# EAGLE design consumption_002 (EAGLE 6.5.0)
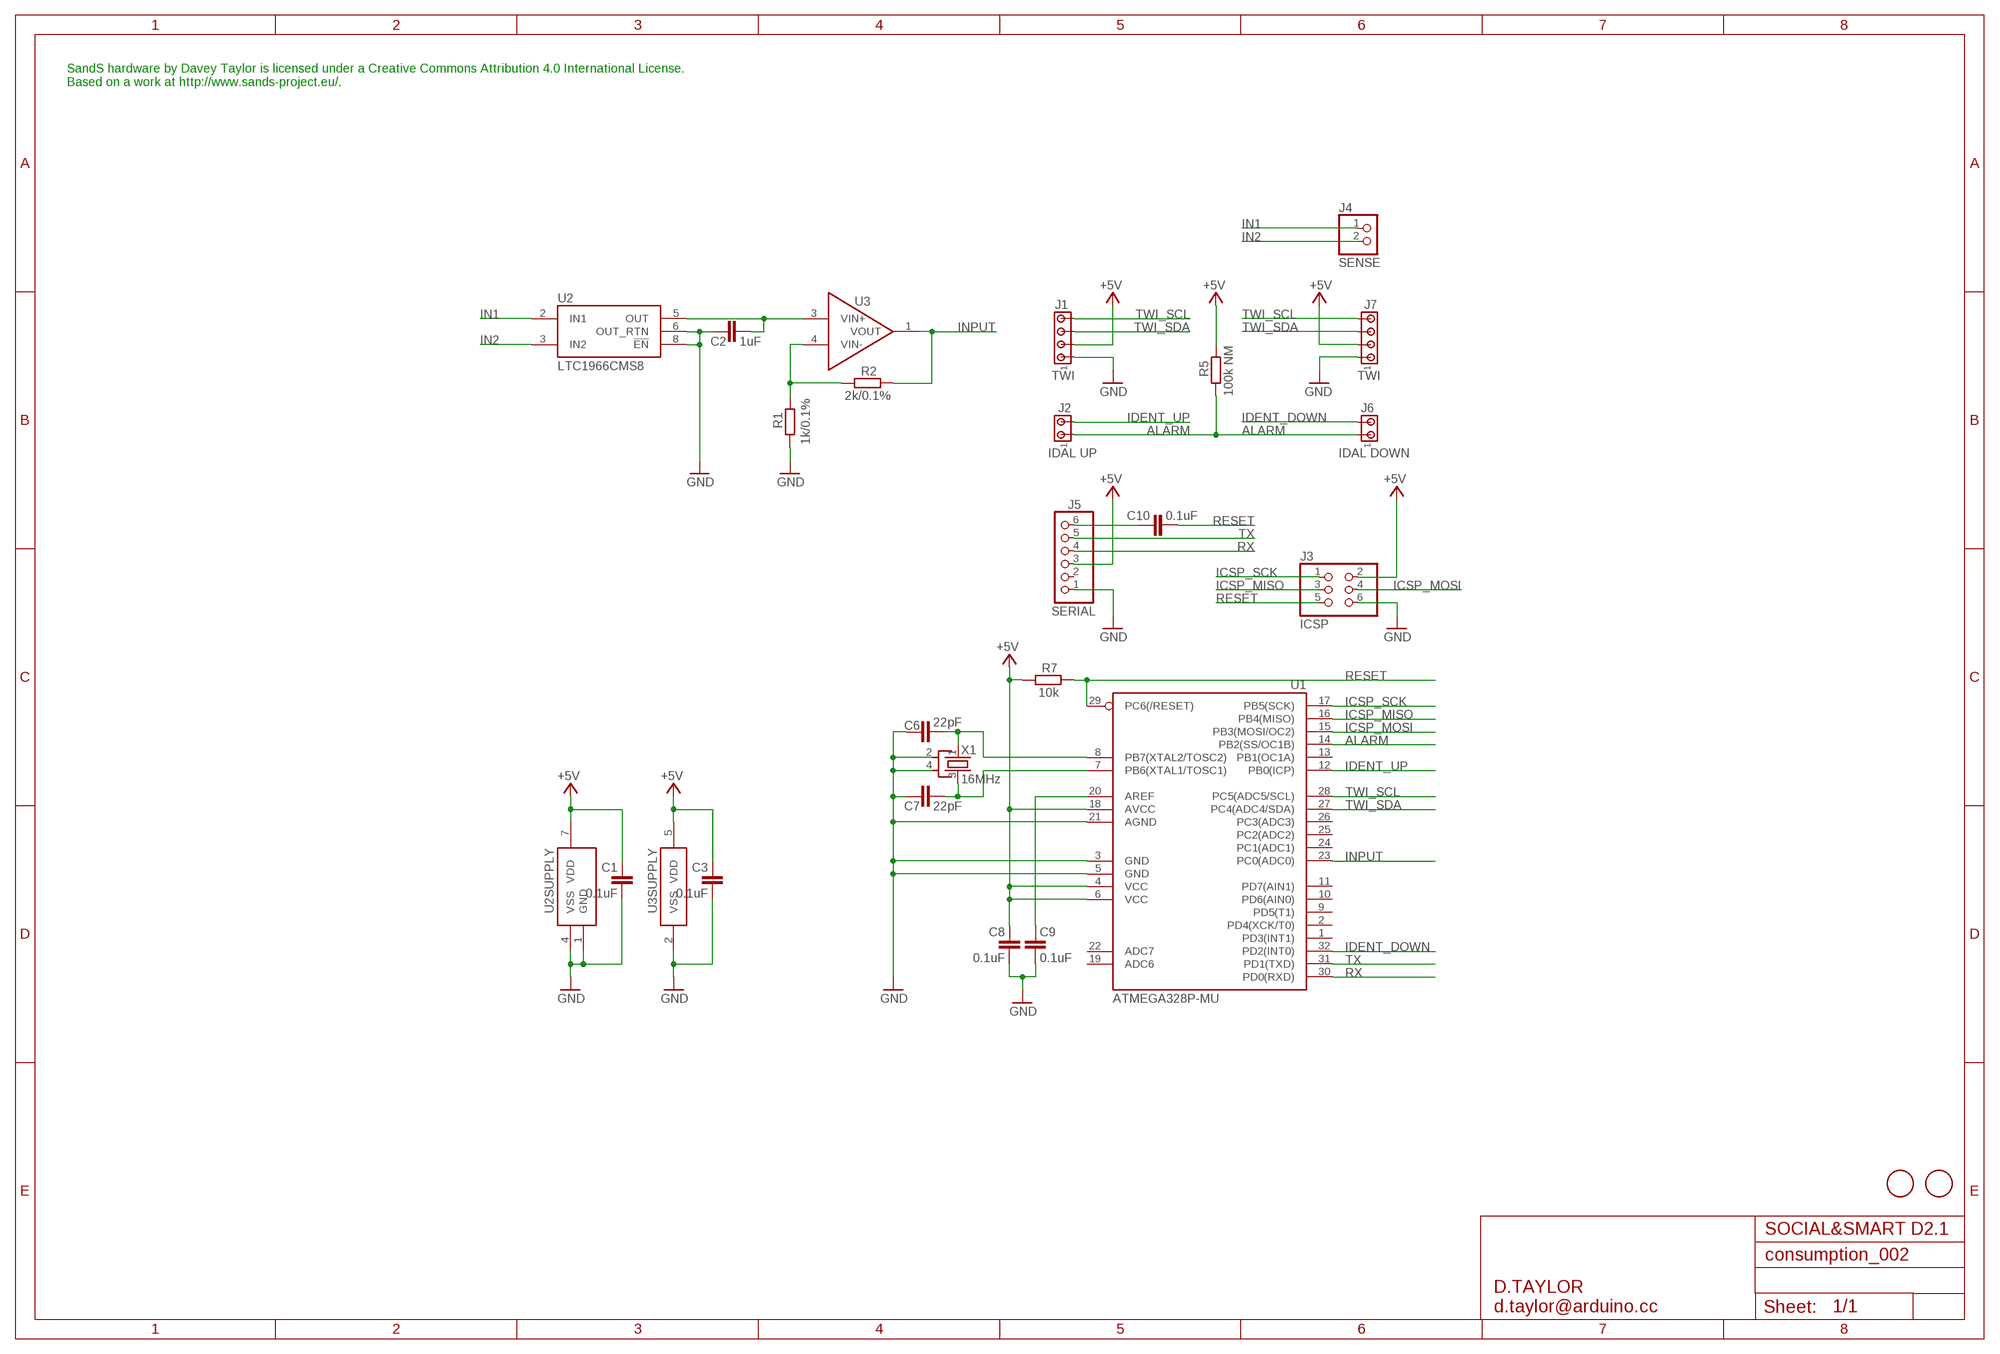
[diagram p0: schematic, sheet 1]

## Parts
C1  0.1uF  C-EUC0603  [C0603]
C2  1uF  C-EUC0603  [C0603]
C3  0.1uF  C-EUC0603  [C0603]
C6  22pF  C-EUC0603  [C0603]
C7  22pF  C-EUC0603  [C0603]
C8  0.1uF  C-EUC0603  [C0603]
C9  0.1uF  C-EUC0603  [C0603]
C10  0.1uF  C-EUC0603  [C0603]
J1  TWI  MTA04-100  [10X04MTA]
J2  IDAL UP  MTA02-100  [10X02MTA]
J3  ICSP  PINHD-2X3  [2X03]
J4  SENSE  MKDS_1,5/2-5,08  [MKDS1,5/2-5,08]
J5  SERIAL  PINHD-1X6  [1X06]
J6  IDAL DOWN  MTA02-100  [10X02MTA]
J7  TWI  MTA04-100  [10X04MTA]
R1  1k/0.1%  R-EU_R0603  [R0603]
R2  2k/0.1%  R-EU_R0603  [R0603]
R5  100k NM  R-EU_R0603  [R0603]
R7  10k  R-EU_R0603  [R0603]
U1  ATMEGA328P-MU  [MLF32-M1-A]
U2  LTC1966CMS8  [MSOP08]
U3  MCP6401T-E/OT  MCP6401-E/OT  [SOT-23-5]
U$5  FIDUCIALMOUNT  [FIDUCIA-MOUNT]
U$6  FIDUCIALMOUNT  [FIDUCIA-MOUNT]
X1  16MHz  CRYSTAL-KX7  [XTAL-3.2-2.5]

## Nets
+5V: C1.1 C3.1 C8.1 J1.2 J3.2 J5.3 J7.2 R5.2 R7.1 U1.4(VCC) U1.6(VCC) U1.18(AVCC) U2.7(VDD) U3.5(VDD)
ALARM: J2.1 J6.1 R5.1 U1.14(PB2(SS/OC1B))
GND: C1.2 C2.1 C3.2 C6.1 C7.1 C8.2 C9.2 J1.1 J3.6 J5.1 J7.1 R1.1 U1.3(GND) U1.5(GND) U1.21(AGND) U2.1(GND) U2.4(VSS) U2.6(OUT_RTN) U2.8(!EN!) U3.2(VSS) X1.2(SH1) X1.4(SH2)
ICSP_MISO: J3.3 U1.16(PB4(MISO))
ICSP_MOSI: J3.4 U1.15(PB3(MOSI/OC2))
ICSP_SCK: J3.1 U1.17(PB5(SCK))
IDENT_DOWN: J6.2 U1.32(PD2(INT0))
IDENT_UP: J2.2 U1.12(PB0(ICP))
IN1: J4.1 U2.2(IN1)
IN2: J4.2 U2.3(IN2)
INPUT: R2.1 U1.23(PC0(ADC0)) U3.1(VOUT)
N$1: C2.2 U2.5(OUT) U3.3(VIN+)
N$2: R1.2 R2.2 U3.4(VIN-)
N$3: C9.1 U1.20(AREF)
N$6: C6.2 U1.8(PB7(XTAL2/TOSC2)) X1.1(X1)
N$7: C7.2 U1.7(PB6(XTAL1/TOSC1)) X1.3(X2)
N$9: C10.1 J5.6
RESET: C10.2 J3.5 R7.2 U1.29(PC6(/RESET))
RX: J5.4 U1.30(PD0(RXD))
TWI_SCL: J1.4 J7.4 U1.28(PC5(ADC5/SCL))
TWI_SDA: J1.3 J7.3 U1.27(PC4(ADC4/SDA))
TX: J5.5 U1.31(PD1(TXD))
Unconnected: J5.2 U1.1(PD3(INT1)) U1.2(PD4(XCK/T0)) U1.9(PD5(T1)) U1.10(PD6(AIN0)) U1.11(PD7(AIN1)) U1.13(PB1(OC1A)) U1.19(ADC6) U1.22(ADC7) U1.24(PC1(ADC1)) U1.25(PC2(ADC2)) U1.26(PC3(ADC3))

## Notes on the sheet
- SandS hardware by Davey Taylor is licensed under a Creative Commons Attribution 4.0 International License.
  Based on a work at http://www.sands-project.eu/.
- SOCIAL&SMART D2.1
- D.TAYLOR
  d.taylor@arduino.cc

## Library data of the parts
C1-C3 C6-C10 = rcl:C-EU: CAPACITOR, European symbol
J1 J7 = con-amp:MTA04-100: AMP connector
J2 J6 = con-amp:MTA02-100: AMP connector
J3 = pinhead:PINHD-2X3: PIN HEADER
J4 = d_taylor:MKDS_1,5/2-5,08: Screw terminal header
J5 = pinhead:PINHD-1X6: PIN HEADER
R1 R2 R5 R7 = rcl:R-EU_: RESISTOR, European symbol
U1 = d_taylor:ATMEGA*: MICROCONTROLLER 8 Kbytes FLASH 1 kbytes SRAM 512 bytes EEPROM USART 6-channel 10 bit ADC 2-channel 8 bit ADC Source: avr.lbr
U2 = d_taylor:LTC1966*MS8: Precision Micropower Delta-Sigma RMS-to-DC Converter
U3 = d_taylor:MCP6401*
U$5 U$6 = SmartPrj:FIDUCIALMOUNT
X1 = d_taylor:CRYSTAL-KX7

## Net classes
1 PWR: width 0.406 mm, clearance 0.254 mm

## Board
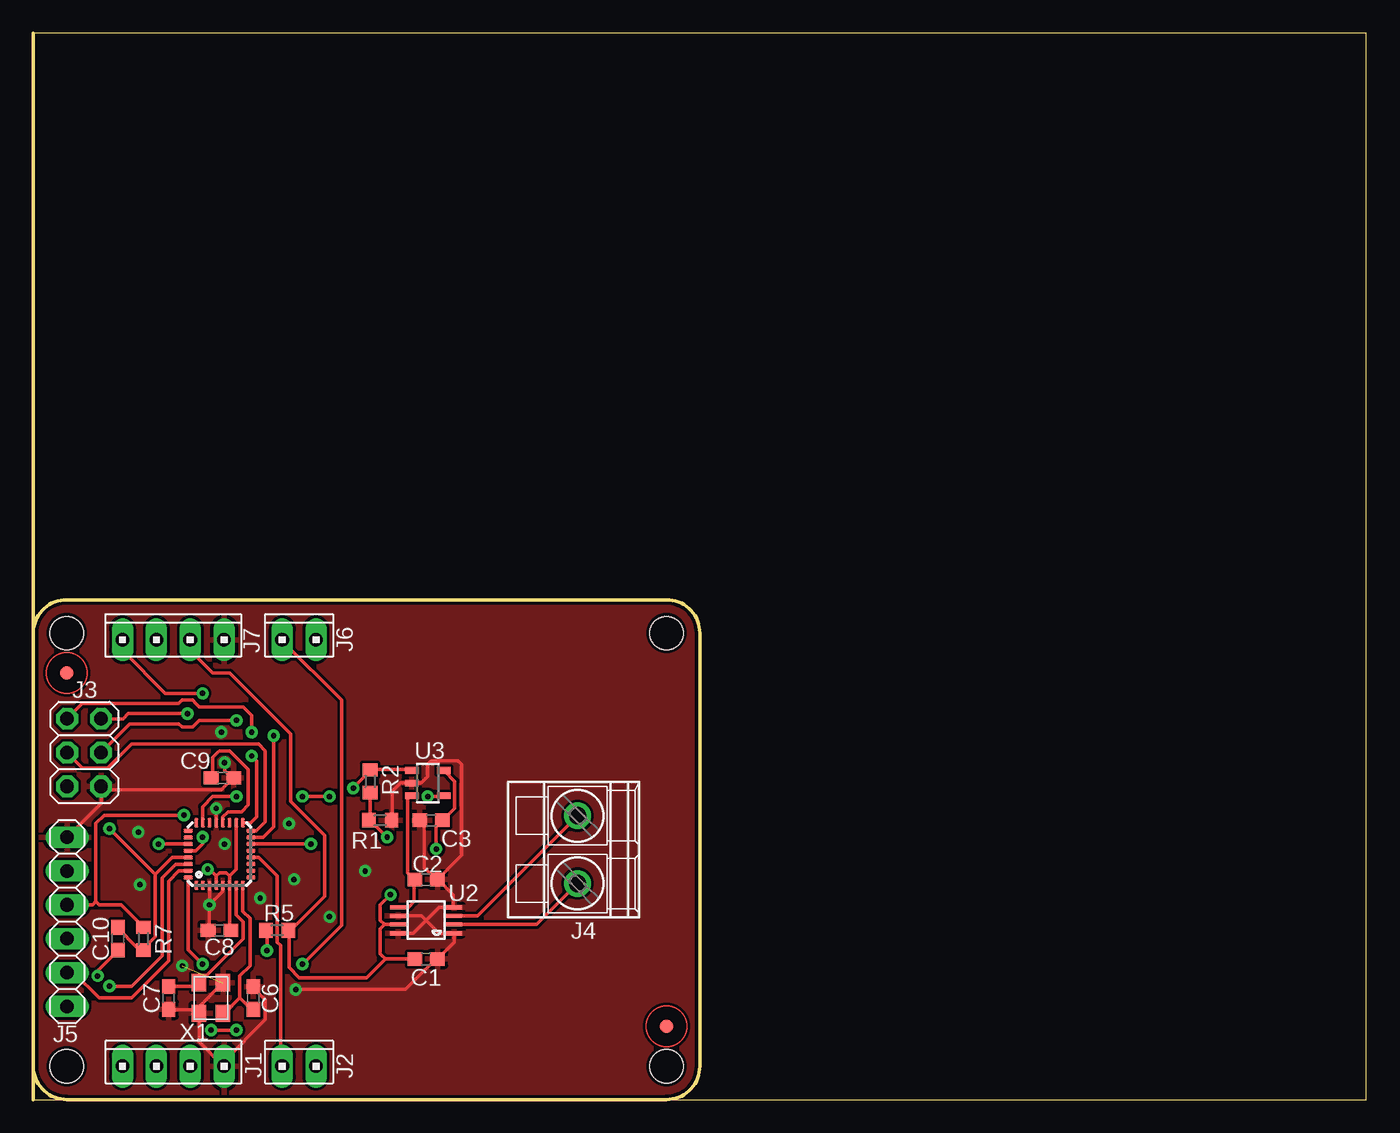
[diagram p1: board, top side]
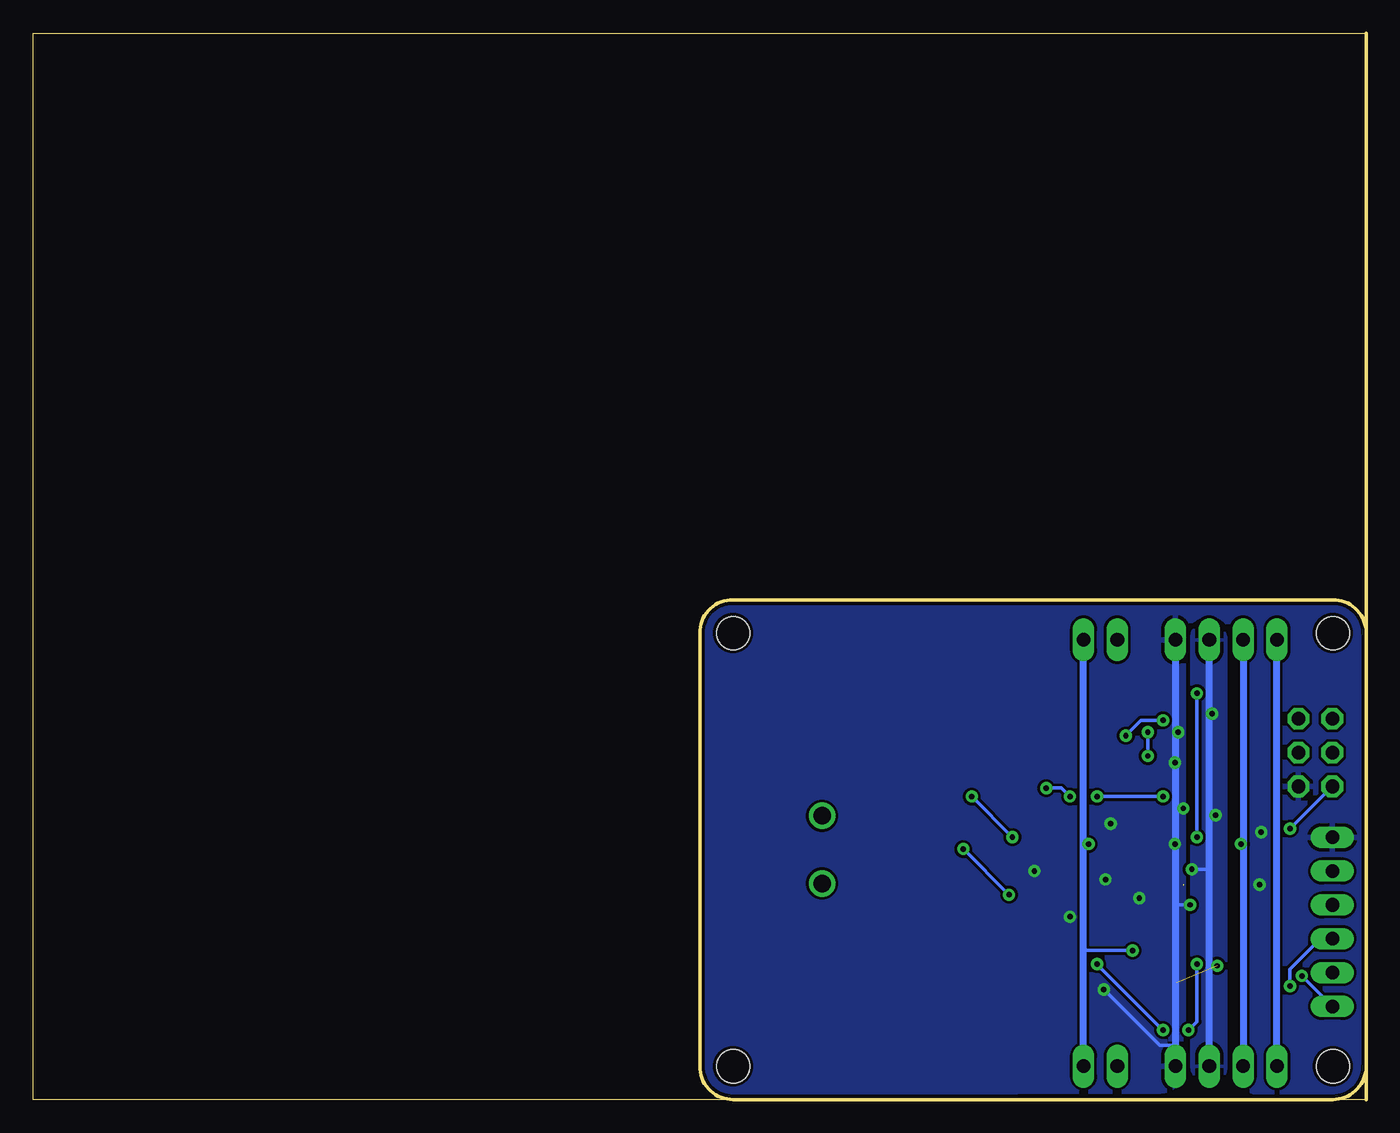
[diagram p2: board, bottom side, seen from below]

Size 100 x 80 mm. Coordinates in mm from the lower left corner, seen from the top.
Outline: 0,35 0,80 100,80 100,0 0,0 0,35
Outline: 0,35 arc-90 2.5,37.5 47.5,37.5 arc-90 50,35 50,2.5 arc-90 47.5,0 2.5,0 arc-90 0,2.5 0,35
Copper layers (1*16): Top 0.035mm / dielectric 1.5mm / Bottom 0.035mm
Design rules "smartprj-mini *": minimum track width 8mil, minimum drill 16mil, track to track 8mil, track to pad 8mil, pad to pad 0.200659375mm, via to via 8mil, smd to smd 4mil, copper to edge 10mil, drill to drill 8mil, minimum pad ring 12mil, minimum via ring 10mil, stop-mask expansion 2mil, vias tented up to drill 20mil, thermal gap 10mil
Holes 2.5 mm at 2.5,35 2.5,2.5 47.5,2.5 47.5,35

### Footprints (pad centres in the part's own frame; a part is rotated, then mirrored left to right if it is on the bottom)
C0603 = smd 1.1 x 1: 1 -0.85,0; 2 0.85,0
10X04MTA = drill 1.016 long: 1 3.81,0; 2 1.27,0; 3 -1.27,0; 4 -3.81,0
10X02MTA = drill 1.016 long: 1 1.27,0; 2 -1.27,0
2X03 = drill 1.016 octagon: 1 -2.54,-1.27; 2 -2.54,1.27; 3 0,-1.27; 4 0,1.27; 5 2.54,-1.27; 6 2.54,1.27
MKDS1,5/2-5,08 = drill 1.3 pad 2: 1 -2.54,0; 2 2.54,0
1X06 = drill 1.016 long: 1 -6.35,0; 2 -3.81,0; 3 -1.27,0; 4 1.27,0; 5 3.81,0; 6 6.35,0
R0603 = smd 1 x 1.1: 1 -0.85,0; 2 0.85,0
MLF32-M1-A = smd 0.7 x 0.3: 1 -2.35,1.75; 2 -2.35,1.25; 3 -2.35,0.75; 4 -2.35,0.25; 5 -2.35,-0.25; 6 -2.35,-0.75; 7 -2.35,-1.25; 8 -2.35,-1.75; 17 2.35,-1.75; 18 2.35,-1.25; 19 2.35,-0.75; 20 2.35,-0.25; 21 2.35,0.25; 22 2.35,0.75; 23 2.35,1.25; 24 2.35,1.75 | smd 0.3 x 0.7: 9 -1.75,-2.35; 10 -1.25,-2.35; 11 -0.75,-2.35; 12 -0.25,-2.35; 13 0.25,-2.35; 14 0.75,-2.35; 15 1.25,-2.35; 16 1.75,-2.35; 25 1.75,2.35; 26 1.25,2.35; 27 0.75,2.35; 28 0.25,2.35; 29 -0.25,2.35; 30 -0.75,2.35; 31 -1.25,2.35; 32 -1.75,2.35
MSOP08 = smd 0.3 x 1.2: 1 -0.976,-2.113; 2 -0.326,-2.113; 3 0.324,-2.113; 4 0.974,-2.113; 5 0.974,2.112; 6 0.324,2.112; 7 -0.326,2.112; 8 -0.976,2.112
SOT-23-5 = smd 0.5 x 1: 1 -0.95,-1.2; 2 0,-1.2; 3 0.95,-1.2; 4 0.95,1.2; 5 -0.95,1.2
FIDUCIA-MOUNT = smd 1.016 x 1.016: P$1 0,0
XTAL-3.2-2.5 = smd 1.3 x 1.1: 1 -1.15,-0.9; 2 1.15,-0.9; 3 1.15,0.9; 4 -1.15,0.9

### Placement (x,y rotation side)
C1  29.46,10.54 0 top
C2  29.46,16.51 180 top
C3  29.84,20.95 180 top
C6  16.51,7.62 270 top
C7  10.16,7.62 90 top
C8  13.97,12.7 180 top
C9  14.2,24.13 0 top
C10  6.35,12.06 90 top
J1  10.5,2.5 0 top
J2  19.94,2.5 0 top
J3  3.81,26.04 270 top
J4  40.83,18.75 90 top
J5  2.54,13.34 270 top
J6  19.94,34.5 0 top
J7  10.5,34.5 0 top
R1  26.04,20.95 180 top
R2  25.27,23.88 270 top
R5  18.29,12.7 0 top
R7  8.26,12.06 270 top
U1  13.97,18.41 90 top
U2  29.46,13.46 90 top
U3  29.59,23.75 270 top
U$5  2.5,32 0 top
U$6  47.5,5.5 0 top
X1  13.34,7.62 90 top

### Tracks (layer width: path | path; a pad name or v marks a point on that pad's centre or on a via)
+5V  (via drill 0.41)  (1 unrouted)
  Top 0.254: U3.5 30.86,24.64 31.62,23.88 31.62,21.84 30.73,20.95 C3.1 30.61,20.95 30.23,20.57 v30.23,18.8 | 26.42,10.54 28.57,10.54 C1.1 | 26.42,10.54 26.16,10.79 26.04,10.92 26.04,11.56 26.04,12.81 26.36,13.14 | 26.42,10.54 25.02,9.14 19.94,9.14 19.18,9.91 19.18,12.45 19.18,12.7 R5.2 19.3,12.7 21.84,15.24 21.84,19.81 19.3,22.35 19.3,27.43 14.73,32 13.46,32 11.81,33.66 11.81,34.42 J7.2 | v26.8,15.37 26.04,14.61 26.04,13.46 26.36,13.14 | J5.3 4.45,14.61 4.7,14.86 | 4.7,14.86 4.95,14.61 6.6,14.61 8.26,12.95 R7.1 | 14.73,16.76 14.73,16.13 U1.6 14.73,16 14.73,12.7 C8.1 | J3.2 6.73,28.57 7.11,28.96 v11.56,28.96 | 4.7,14.86 4.7,20.7 5.33,21.34 v11.3,21.34 | U2.7 26.36,13.14 | 13.72,16.13 13.72,16.76 | 13.72,16.76 13.97,17.02 14.48,17.02 14.73,16.76 | v13.08,17.27 13.21,17.27 13.72,16.76 | U1.18 15.22,17.25 14.73,16.76
  Bottom 0.203: 11.94,17.27 11.77,17.27
  Bottom 0.254: v26.8,15.37 v30.23,18.8 | v11.56,28.96 11.77,28.96 | 11.94,17.27 v13.08,17.27 | v11.3,21.34 11.68,21.34 11.77,21.34
  Bottom 0.508: J1.2 11.77,17.27 11.77,21.34 11.77,28.96 J7.2
  pour Bottom: 13.08,34.67 arc90 11.94,35.81 11.81,35.81 arc90 10.54,34.54 10.54,2.54 10.54,2.41 arc90 11.68,1.27 11.81,1.27 arc90 13.08,2.54
ALARM  (via drill 0.41)
  Top 0.254: v20.83,19.18 16.38,19.18 U1.14 | v17.53,11.18 17.53,12.7 R5.1
  Bottom 0.203: 21.08,11.18 21.21,11.18
  Bottom 0.254: v20.83,19.18 21.21,19.18 | 21.08,11.18 v17.53,11.18
  Bottom 0.508: J2.1 21.21,11.18 21.21,19.18 J6.1
GND  (via drill 0.41)  (1 unrouted)
  Top 0.254: 5.08,23.24 14.1,23.24 14.99,24.13 C9.2 14.86,24.13 14.35,24.64 v14.35,25.27 | 5.08,23.24 J3.6 5.08,23.24 | J5.1 5.08,22.23 5.08,23.24 | 30.35,10.54 C1.2 | 31.5,12.45 U2.1 | R1.1 26.92,20.95 26.92,23.11 27.56,23.75 28.32,23.75 U3.2 28.45,23.75 29.08,23.75 29.59,24.26 29.59,25.15 29.84,25.4 30.1,25.4 31.75,25.4 31.88,25.4 32.13,25.15 32.13,19.56 32.13,18.33 C2.1 | 30.35,16.51 C2.1 | C3.2 29.08,20.95 29.34,20.57 29.34,17.4 29.65,17.08 30.23,16.51 C2.1 | C8.2 13.21,12.7 v13.21,14.61 | 14.22,16 U1.5 14.22,15.62 v13.21,14.61 | v13.72,21.84 13.72,20.83 U1.21 | X1.4 12.45,6.35 12.45,4.32 14.22,2.54 J1.1 14.35,2.92 17.4,5.97 17.4,7.49 16.51,8.38 C6.1 | 12.32,6.73 10.16,6.73 C7.1 | 12.32,6.73 12.32,6.48 X1.4 | 12.32,6.73 12.32,6.86 14.22,8.76 X1.2 | 12.32,6.73 X1.4 | v19.68,8.26 27.94,8.26 30.23,10.54 C1.2 | C2.1 30.35,16.51 | 30.35,16.51 31.5,15.37 31.5,14.52 U2.4 30.44,14.44 29.46,13.46 | 29.46,13.46 30.44,12.49 U2.1 | U2.8 28.49,12.49 29.46,13.46 | U2.6 29.14,13.79 29.46,13.46 | C1.2 31.58,11.8 U2.1 | U1.3 v13.22,14.62 v13.21,14.61
  Bottom 0.203: 14.48,4.06 14.31,4.06
  Bottom 0.254: v13.72,21.84 14.1,21.84 14.31,21.84 | v13.21,14.61 14.1,14.61 14.31,14.61 | v19.68,8.26 15.49,4.06 14.48,4.06 | v14.35,25.27 14.31,25.27
  Bottom 0.508: J7.1 14.31,25.27 14.31,21.84 14.31,14.61 14.31,4.06 J1.1
  other vias: 24.89,17.14 19.56,16.51 17.02,15.11 19.18,20.7 8,16.13 14.35,19.18 11.18,10.03 22.23,13.72 14.1,27.56 7.87,20.07
  pour Top: 0.5,35 arc-90 2.5,37 47.5,37 arc-90 49.5,35 49.5,2.5 arc-90 47.5,0.5 2.5,0.5 arc-90 0.5,2.5
  pour Bottom: 0.5,35 arc-90 2.5,37 47.5,37 arc-90 49.5,35 49.5,2.5 arc-90 47.5,0.5 15.49,0.64 arc-90 13.72,2.41 13.72,34.42 arc90 11.81,36.45 arc90 9.91,34.54 9.91,2.54 arc-90 7.87,0.5 2.5,0.5 arc-90 0.5,2.5
ICSP_MISO
  Top 0.254: J3.3 3.68,24.89 5.59,24.89 7.37,26.67 16.89,26.67 17.4,26.16 17.4,20.83 16.74,20.16 U1.16
ICSP_MOSI  (via drill 0.41)
  Top 0.254: v18.03,27.3 18.03,20.45 17.25,19.66 U1.15 | v15.24,28.45 12.45,28.45 11.94,27.94 11.18,27.94 10.92,28.19 7.24,28.19 J3.4
  Bottom 0.254: v18.03,27.3 16.89,28.45 v15.24,28.45
ICSP_SCK  (via drill 0.41)
  Top 0.254: 16.76,25.4 v16.38,25.78 16.76,25.4 | v16.38,27.56 16.38,28.83 15.75,29.46 12.45,29.46 12.19,29.72 11.94,29.97 11.18,29.97 10.92,29.72 3.68,29.72 J3.1 | U1.17 16.32,20.77 16.76,21.21 16.76,25.4
  Bottom 0.254: v16.38,27.56 v16.38,25.78
IDENT_DOWN  (via drill 0.41)
  Top 0.254: v15.24,5.21 v13.34,5.21 | v20.19,10.16 23.11,13.08 23.11,29.97 18.67,34.42 J6.2 | U1.32 11.62,11.24 v12.7,10.16
  Bottom 0.254: v13.34,5.21 12.7,5.84 v12.7,10.16 | v20.19,10.16 v15.24,5.21
IDENT_UP
  Top 0.254: U1.12 16.38,18.16 16.89,18.16 18.29,16.76 18.29,11.81 18.54,11.56 18.54,2.67 18.67,2.54 J2.2
IN1
  Top 0.254: U2.2 37.75,13.14 J4.1
IN2
  Top 0.254: U2.3 33.32,13.79 J4.2
INPUT  (via drill 0.41)
  Top 0.254: v15.24,22.73 13.46,22.73 12.7,21.97 12.7,20.83 U1.23 | v22.23,22.73 v20.19,22.73 | v24,23.37 25.27,24.64 R2.1 25.27,24.77 28.32,24.77 U3.1
  Bottom 0.254: v20.19,22.73 v15.24,22.73 | v22.23,22.73 22.86,23.37 v24,23.37
N$1
  Top 0.254: U3.3 28.07,22.61 28.07,17.02 28.57,16.51 C2.2 28.57,16.47 28.57,14.86 28.15,14.44 U2.5
N$2  (via drill 0.41)
  Top 0.254: v29.59,22.73 30.73,22.73 U3.4 | 25.27,20.95 v26.54,19.68 | 25.27,20.95 R1.2 25.27,20.95 | 25.27,20.95 25.27,22.99 R2.2
  Bottom 0.254: v26.54,19.68 v29.59,22.73
N$3
  Top 0.254: U1.20 14.22,20.83 14.22,21.21 14.61,21.59 15.62,21.59 16.13,22.1 16.13,24.77 14.73,26.16 13.97,26.16 13.84,26.04 13.46,25.65 13.46,24.13 C9.1
N$6
  Top 0.254: 15.49,7.62 15.49,9.27 16.26,10.03 16.26,13.59 15.72,14.12 U1.8 | 15.49,7.62 16.26,6.86 C6.2 | 15.49,7.62 14.35,6.48 X1.1
N$7
  Top 0.254: C7.2 10.16,8.51 12.32,8.51 12.32,8.76 X1.3 15.75,12.06 15.75,13.34 15.22,13.86 U1.7
N$9  (via drill 0.41)
  Top 0.254: v4.83,9.27 4.83,9.65 6.35,11.18 C10.1
  Bottom 0.254: J5.6 v4.83,9.27
RESET  (via drill 0.41)
  Top 0.254: 9.14,16.89 9.14,12.19 8.26,11.3 R7.2 8.26,11.43 7.75,11.43 6.35,12.83 C10.2 | U1.29 11.56,18.16 10.41,18.16 9.14,16.89 | 9.14,16.89 v5.71,20.32
  Bottom 0.254: v5.71,20.32 J3.5
RX  (via drill 0.41)
  Top 0.254: v5.71,8.51 7.37,8.51 9.65,10.79 9.65,16.64 10.67,17.65 11.56,17.65 U1.30
  Bottom 0.254: v5.71,8.51 5.71,9.78 3.43,12.06 3.3,12.06 J5.4
TWI_SCL  (via drill 0.41)
  Top 0.254: v12.7,19.68 12.7,19.18 12.19,18.67 11.68,18.67 U1.28 | v12.7,30.48 9.91,30.48 6.73,33.66 J7.4
  Bottom 0.254: v12.7,30.48 v12.7,19.68
  Bottom 0.508: J1.4 J7.4
TWI_SDA  (via drill 0.41)
  Top 0.254: v9.4,19.18 11.56,19.18 U1.27
  Bottom 0.203: v9.4,19.18 9.23,19.18
  Bottom 0.508: J7.3 9.23,19.18 J1.3
TX
  Top 0.254: J5.5 3.05,9.53 4.95,7.62 7.37,7.62 10.16,10.41 10.16,16.38 10.92,17.14 11.56,17.14 U1.31

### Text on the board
tDocu: TWI | IDAL-D | ICSP | SENSOR | SERIAL | TWI | IDAL-U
